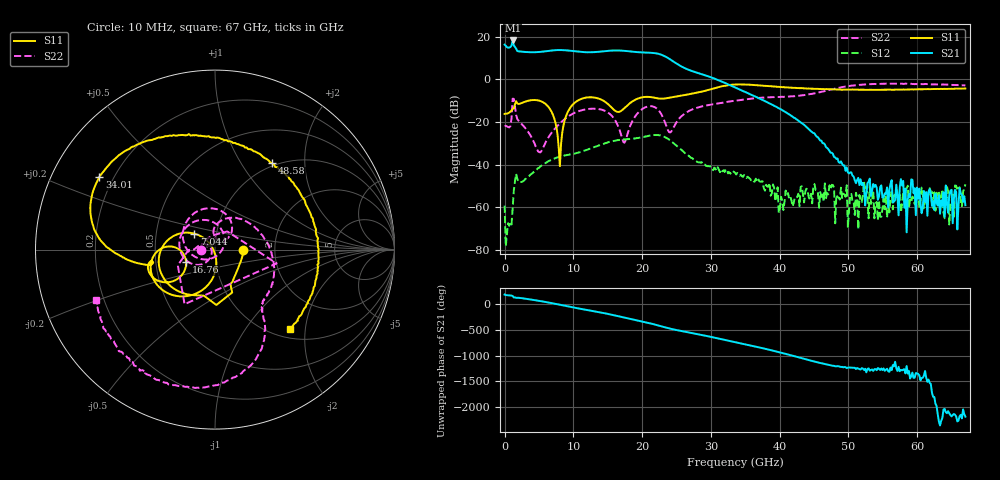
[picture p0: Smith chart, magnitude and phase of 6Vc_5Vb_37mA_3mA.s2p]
! MARKI MICROWAVE INC.
! Date:  05/05/2020
! Model Number:  APM-7099CH
! Description:  2-port Small Signal S-parameter data for APM-7099CH
! Frequency Range:  10 MHz to 67 GHz
! Port Configuration:  PORT 1: Input
!  PORT 2: Output
! Bias Condition: Vc = +6V, Vb = +5V
! APM-7099CH s2p files are only valid for small signal conditions (below -5 dBm input power)
!S2P File: Measurements: Mag<S11> Ang<S11>, Mag<S21> Ang<S21>, Mag<S12> Ang<S12>, Mag<S22> Ang<S22>!row 1
# Hz S  dB  R 50
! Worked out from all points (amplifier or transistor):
!   401 points, 10 MHz to 67 GHz, reference 50 ohm
!   highest |S21| = 18.2 dB at 1.182 GHz (marker M1)
!   |S21| within 3 dB of that: 874.4 MHz to 1.497 GHz (622.4 MHz wide, 52.5 % of centre)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
!   unconditionally stable (mu >= 1): start of sweep to end of sweep
!   at 11.06 GHz: K = 4.94, MAG = 13.6 dB, |S12| = -34.1 dB
!   at 33.51 GHz: K = 46.01, MAG = 0.3 dB, |S12| = -43.8 dB
!   at 67 GHz: K = 38709.29, MAG = -53.8 dB, |S12| = -49.2 dB
!   S11 on the Smith chart (normalised r, x): 10 MHz: 1.37, -0.01; 7.044 GHz: 0.78, +0.14; 16.76 GHz: 0.72, -0.10; 34.01 GHz: 0.15, +0.28; 48.58 GHz: 0.96, +1.38; 67 GHz: 1.17, -1.66
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1e7  -16.20 -0.9  16.25 178.7  -59.20 -48.8  -21.92 -178.3
1.182325e9  -13.83 -61.3  18.23 149.4  -60.47 80.7  -9.07 -12.6
1.68475e9  -10.21 -88.6  14.36 115.4  -44.29 -79.1  -16.64 -179.2
4.36435e9  -9.68 -156.4  12.70 70.8  -43.03 -162.9  -30.05 151.5
7.04395e9  -16.66 142.4  13.58 8.1  -37.38 135.5  -24.17 -121.3
9.221125e9  -15.12 -97.0  13.51 -51.0  -35.35 86.0  -17.48 -140.5
1.123082e10  -9.07 -135.0  12.83 -101.2  -33.85 49.4  -14.46 -173.4
1.441285e10  -10.10 -179.6  13.15 -178.7  -30.18 -14.5  -14.53 120.0
1.67575e10  -15.14 -157.3  13.51 113.8  -28.35 -72.5  -24.05 33.6
1.826478e10  -11.08 -142.3  13.09 69.2  -27.93 -109.4  -21.83 -136.9
1.993952e10  -8.48 -155.1  12.62 20.5  -27.17 -150.0  -14.12 155.8
2.127932e10  -8.33 -166.7  12.44 -21.4  -26.26 172.3  -12.55 106.0
2.245165e10  -9.00 -169.4  11.88 -62.6  -26.16 132.4  -14.70 61.8
2.379145e10  -8.70 -166.8  9.94 -110.6  -27.91 84.4  -24.07 53.2
2.513125e10  -7.95 -168.0  7.14 -150.9  -31.46 46.2  -19.53 94.4
2.88157e10  -5.64 -175.9  2.28 114.8  -39.42 -3.1  -12.62 42.2
3.3505e10  -2.43 152.4  -3.78 -19.7  -43.75 -60.9  -10.00 -3.2
3.400742e10  -2.38 147.9  -4.51 -33.9  -44.46 -75.2  -9.82 -7.4
4.472582e10  -4.37 79.2  -24.73 -24.5  -58.12 -33.6  -6.76 -54.1
4.857775e10  -4.80 56.7  -38.78 -128.0  -55.46 -58.8  -3.96 -67.8
5.594665e10  -4.84 12.0  -51.71 126.4  -62.35 -135.9  -2.06 -109.8
6.7e10  -4.30 -46.7  -58.99 -20.5  -49.20 -23.0  -2.84 -156.9
